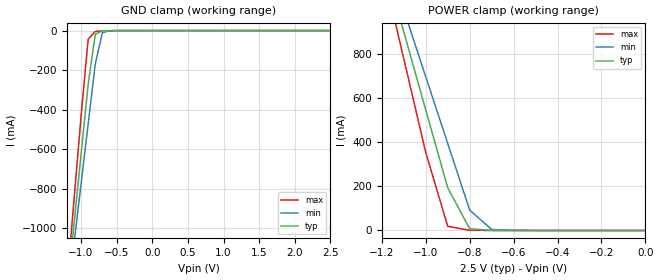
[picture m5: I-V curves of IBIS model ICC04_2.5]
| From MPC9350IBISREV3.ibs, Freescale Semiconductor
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|   ICC04_2.5: LVCMOS INPUT MODEL WITH A 25K PULLDOWN RESISTOR
[Model]   ICC04_2.5
Model_type  Input
Vinh   =  1.7
Vinl   =  0.7
C_comp   4pF   4pF   4pF
[Temperature Range] 55   110   0
[Voltage Range]   2.5   2.25   2.75
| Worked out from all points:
|   GND clamp passes 1 mA (typ) near -0.64 V on its own axis
|   POWER clamp passes 1 mA (typ) near -0.71 V on its own axis
[GND Clamp]
-2.5V     -5.969A    -5.351A    -6.849A
-1.2V     -1.34A     -1.387A    -1.291A
-1.1V     -983.9mA   -1.082A    -863.3mA
-1V       -628.2mA   -777.7mA   -436mA
-900mV    -272.7mA   -473.4mA   -43.64mA
-800mV    -18.4mA    -169.2mA   -4.102mA
-700mV    -1.832mA   -10.56mA   -1.775mA
-600mV    -494uA     -870uA     -572.7uA
2.5V      101.9uA    108uA      96.41uA
[POWER Clamp]
-2.5V     5.872A     5.257A     6.751A
-1.2V     1.258A     1.306A     1.207A
-1.1V     902.9mA    1.003A     780.7mA
-1V       548.4mA    699mA      354.7mA
-900mV    194.1mA    395.6mA    19.08mA
-800mV    7.923mA    92.56mA    770.6uA
-700mV    390.8uA    4.657mA    126.6uA
-600mV    37.06uA    265uA      13.73uA
0V        142.9pA    662pA      21.65pA
